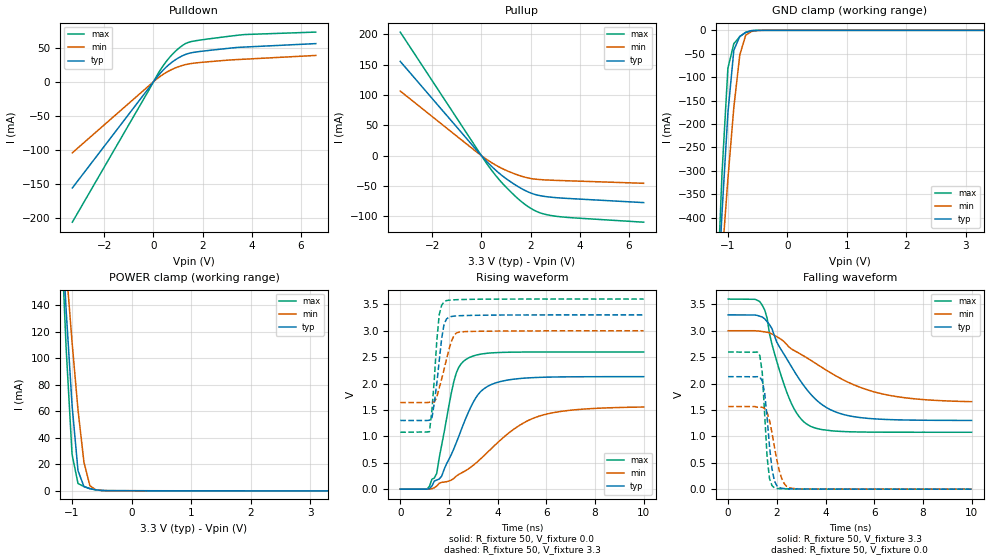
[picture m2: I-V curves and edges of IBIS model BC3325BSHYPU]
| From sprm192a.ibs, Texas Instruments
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[Model]   BC3325BSHYPU
Model_type   I/O
Vinh = 2.00
Vinl = 0.80
Enable   Active-Low
Polarity   Non-Inverting
| signals   A, GZ, Y
Vmeas = 1.5
|   typ   min   max
C_comp   1.4592p   1.4336p   1.5063p
|   typ   min   max
[Temperature Range]   25   -40   125
|   typ   min   max
[Voltage Range]   3.30V   3.00V   3.60V
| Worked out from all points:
|   slope of the pulldown table from 0 to 0.495 V, typ, clamps not added: 24 ohm
|   slope of the pullup table from 0 to 0.495 V, typ, clamps not added: 23.8 ohm
|   GND clamp passes 1 mA (typ) near -0.60 V on its own axis
|   POWER clamp passes 1 mA (typ) near -0.64 V on its own axis
|   rising waveform, R_fixture 50, V_fixture 0.0: 20-80 % time 1.22ns typ, 2.5ns min, 652ps max; typ from 0 V to 2.13 V
|   falling waveform, R_fixture 50, V_fixture 3.3: 20-80 % time 1.69ns typ, 3.02ns min, 994ps max; typ from 3.3 V to 1.3 V
|   rising waveform, R_fixture 50, V_fixture 3.3: 20-80 % time 302ps typ, 455ps min, 243ps max; typ from 1.3 V to 3.3 V
|   falling waveform, R_fixture 50, V_fixture 0.0: 20-80 % time 265ps typ, 404ps min, 205ps max; typ from 2.13 V to 0 V
[Pulldown]
|   Voltage   I(typ)   I(min)   I(max)
-3.3V     -155.6mA   -104.1mA   -205.6mA
200mV     9.244mA    5.866mA    12.7mA
600mV     24.13mA    15.28mA    33.3mA
800mV     29.87mA    18.87mA    41.37mA
1.1V      36.63mA    23.02mA    51.08mA
1.3V      39.97mA    25.04mA    55.82mA
1.6V      42.83mA    27mA       59.28mA
3.5V      50.44mA    32.65mA    68.4mA
6.6V      55.85mA    38.51mA    72.72mA
[GND_clamp]
|   Voltage   I(typ)   I(min)   I(max)
-3.3V     -6.387A    -4.811A    -8.304A
-1.2V     -636.8mA   -670.5mA   -623.6mA
-1.1V     -392.8mA   -489.7mA   -308.9mA
-1V       -176.9mA   -317.9mA   -81.09mA
-900mV    -42.26mA   -164.3mA   -28.41mA
-800mV    -12.97mA   -52.52mA   -13.55mA
-700mV    -4.67mA    -10.2mA    -3.941mA
-600mV    -902.1uA   -2.291mA   -447.8uA
-400mV    -4.618uA   -49.36uA   -472.1nA
3.3V      177.6pA    1.907uA    44.41pA
[Pullup]
|   Voltage   I(typ)   I(min)   I(max)
-3.3V     155.5mA    106.5mA    203.8mA
-200mV    9.303mA    6.23mA     12.42mA
300mV     -13.07mA   -8.543mA   -17.75mA
600mV     -24.68mA   -16mA      -33.64mA
900mV     -34.77mA   -22.33mA   -47.63mA
1.4V      -48.8mA    -30.78mA   -67.76mA
1.7V      -55.89mA   -34.78mA   -78.18mA
2V        -61.53mA   -37.68mA   -86.69mA
2.3V      -65.31mA   -39.22mA   -93.01mA
2.9V      -68.84mA   -40.61mA   -99.22mA
3.7V      -71.03mA   -41.73mA   -102.5mA
6.6V      -77.47mA   -45.64mA   -109.8mA
[POWER_clamp]
|   Voltage   I(typ)   I(min)   I(max)
-3.3V     2.113A     1.594A     2.744A
-1.2V     217.7mA    228.8mA    213mA
-1.1V     136.9mA    169.1mA    108.2mA
-1V       64.54mA    112.3mA    27.47mA
-900mV    15.16mA    60.94mA    5.443mA
-800mV    3.082mA    21.51mA    3.145mA
-700mV    1.489mA    3.764mA    1.661mA
-600mV    649.3uA    707.8uA    623.9uA
-500mV    185.1uA    173.8uA    140.5uA
3.3V      -108.3uA   -68.06uA   -162.1uA
[Ramp]
|   I(typ)   I(min)   I(max)
dV/dt_r   1.278/1.224n   0.933/2.496n   1.559/0.649n
dV/dt_f   1.199/1.691n   0.806/3.021n   1.513/0.994n
[Rising Waveform]
R_fixture = 50
V_fixture = 0.0
|  pu_on
|  TIME   V(typ)   V(min)   V(max)
0s        3nV        16nV       2nV
1.1ns     -156.7uV   -270.2uV   2.656mV
1.5ns     172.5mV    58.53mV    298.7mV
1.7ns     244.2mV    128.6mV    829.3mV
2.2ns     762.3mV    202mV      2.035V
2.4ns     994.3mV    278.9mV    2.304V
2.8ns     1.457V     384mV      2.484V
3.6ns     1.949V     704.6mV    2.575V
5.6ns     2.115V     1.366V     2.597V
10ns      2.131V     1.555V     2.598V
[Falling Waveform]
R_fixture = 50
V_fixture = 3.3
V_fixture_min = 3.0
V_fixture_max = 3.6
|  pd_on
|  TIME   V(typ)   V(min)   V(max)
0s        3.3V       3V         3.6V
1.4ns     3.261V     2.986V     3.482V
1.6ns     3.172V     2.972V     3.241V
1.9ns     2.906V     2.915V     2.576V
2.5ns     2.397V     2.69V      1.729V
2.9ns     2.099V     2.577V     1.383V
3.4ns     1.794V     2.439V     1.187V
5.2ns     1.37V      1.969V     1.085V
7.1ns     1.312V     1.741V     1.078V
10ns      1.302V     1.657V     1.078V
[Rising Waveform]
R_fixture = 50
V_fixture = 3.3
V_fixture_min = 3.0
V_fixture_max = 3.6
|  pd_off
|  TIME   V(typ)   V(min)   V(max)
0s        1.301V     1.641V     1.078V
1.2ns     1.306V     1.646V     1.089V
1.3ns     1.342V     1.649V     1.489V
1.5ns     1.993V     1.741V     2.799V
1.6ns     2.423V     1.914V     3.302V
1.7ns     2.844V     2.083V     3.481V
1.8ns     3.122V     2.267V     3.549V
2.1ns     3.27V      2.798V     3.583V
2.4ns     3.284V     2.973V     3.589V
10ns      3.3V       3V         3.6V
[Falling Waveform]
R_fixture = 50
V_fixture = 0.0
|  pu_off
|  TIME   V(typ)   V(min)   V(max)
0s        2.131V     1.565V     2.598V
1.3ns     2.125V     1.554V     2.53V
1.4ns     2.049V     1.551V     2.211V
1.5ns     1.825V     1.527V     1.412V
1.6ns     1.355V     1.45V      610mV
1.7ns     803.6mV    1.298V     198.7mV
1.9ns     156.8mV    801.9mV    24.84mV
2.2ns     16.98mV    202.5mV    7.255mV
2.6ns     6.073mV    17.47mV    3.352mV
10ns      2.377uV    59.51uV    381nV
